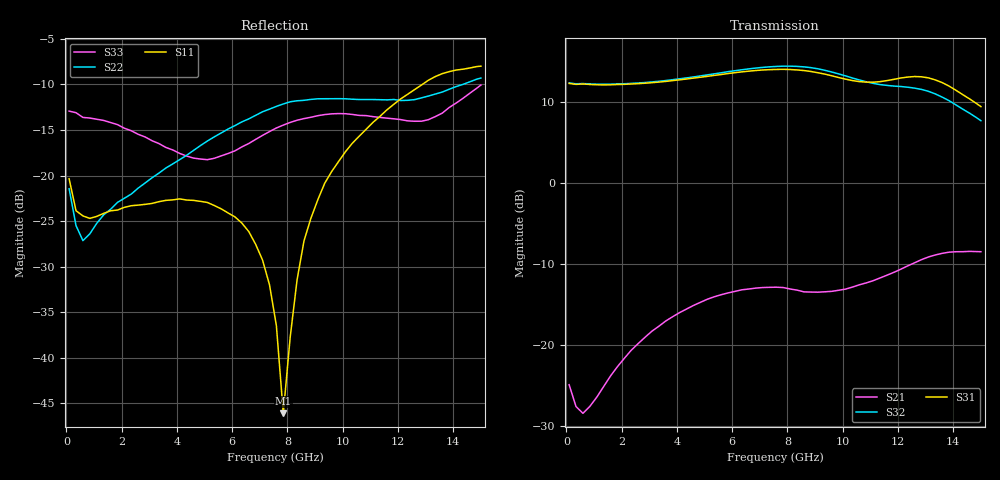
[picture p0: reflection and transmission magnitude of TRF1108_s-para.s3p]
! Created Fri Oct  4 19:43:45 2024
# hz S ri R 50
! 3 Port Network Data from SP1.SP block
! freq  reS11  imS11  reS12  imS12  reS13  imS13
!  reS21  imS21
!  reS22  imS22  reS23  imS23
!  reS31  imS31  reS32  imS32
!  reS33  imS33
! Terminal data exported
! Port[1] = INP
! Port[2] = INM
! Port[3] = OUT
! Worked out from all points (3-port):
!   61 points, 100 MHz to 15 GHz, reference 50 ohm
!   strongest paths, dB at 100 MHz, 3.85 GHz, 7.6 GHz, 11.35 GHz, 15 GHz:
!     S31: 12.3, 12.6, 14.0, 12.5, 9.4
!     S32: 12.3, 12.7, 14.4, 12.1, 7.7
!     S21: -24.9, -16.5, -12.9, -11.7, -8.5
!   lowest |S11| = -46.1 dB at 7.85 GHz (marker M1), VSWR 1.01, Z = 50.5 - j0.0535 ohm
!   |S11| at or under -10 dB: start of sweep to 12.88 GHz
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1e8  -0.0957 0.00796  0.1238 -0.000211  0.00312 -0.000554
     -0.0565 0.00701  0.0847 -0.000268  0.00323 0.00202
     4.098 -0.2731  -4.125 0.278  -0.2256 0.011
2.6e9  -0.0587 0.0359  0.0795 -0.0193  0.00212 0.00151
       0.00634 0.102  0.00656 -0.0851  0.000667 0.000886
       -0.467 -4.067  0.572 4.093  -0.0965 0.1381
4.85e9  -0.0247 0.0678  0.00299 0.0119  0.00446 0.00136
        0.0945 0.1572  -0.1305 -0.0656  0.00294 0.000561
        -4.482 0.165  4.555 -0.3609  -0.042 0.1159
6.35e9  0.00951 0.054  -0.0295 0.1061  0.00559 6.01e-05
        0.1634 0.146  -0.1936 0.0369  0.00328 -0.000807
        -2.159 4.331  1.965 -4.583  -0.0503 0.1346
7.6e9  0.0104 0.0109  0.00664 0.2214  0.00578 -0.00193
       0.1988 0.1104  -0.1854 0.1521  0.00311 -0.00132
       2.347 4.426  -2.803 -4.414  -0.0335 0.1794
7.85e9  0.00493 -0.00053  0.0252 0.2462  0.00612 -0.00216
        0.2022 0.1016  -0.1742 0.1754  0.00272 -0.00116
        3.163 3.893  -3.643 -3.777  -0.0248 0.1877
9.1e9  -0.073 -0.0104  0.1863 0.3105  0.00508 -0.00375
       0.1955 0.0819  -0.0796 0.2516  0.00165 -0.00265
       4.762 -0.4386  -4.936 1.107  0.0323 0.2107
1.11e10  -0.1428 0.1345  0.4238 0.1593  0.00315 -0.00564
         0.2324 0.0905  0.0563 0.2553  0.000384 -0.0019
         0.262 -4.171  0.7581 4.04  0.1078 0.1809
1.31e10  -0.0247 0.3326  0.4298 -0.1096  0.000957 -0.00621
         0.348 0.03  0.1327 0.2388  0.00195 -0.00185
         -4.445 0.0779  3.597 -0.743  0.1119 0.169
1.5e10  0.2538 0.3073  0.287 -0.2296  -0.000187 -0.00781
        0.3403 -0.1606  0.2594 0.2245  0.00257 -0.00357
        0.3651 2.935  -0.4774 -2.372  0.1956 0.2456
